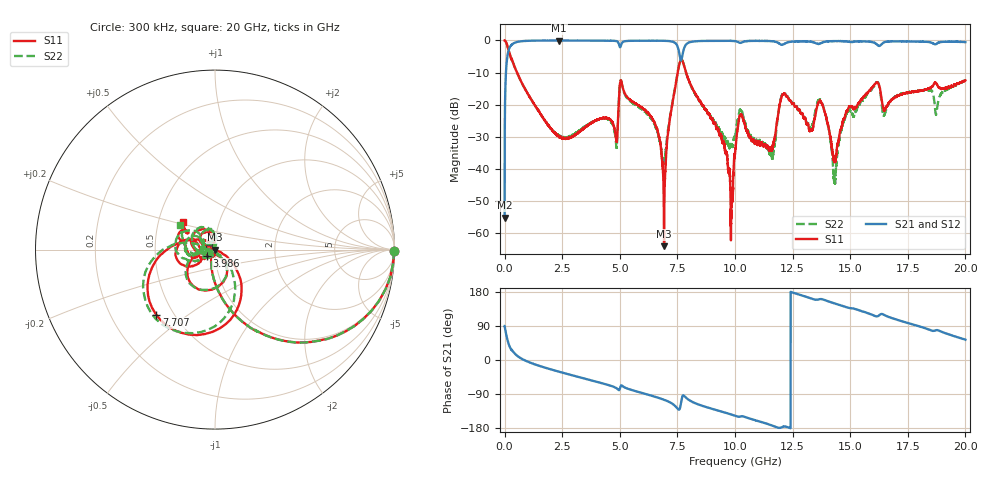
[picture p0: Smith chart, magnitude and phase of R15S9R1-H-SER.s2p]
!{R15S9R1}
!Johanson Technology Inc.
!www.johansontechnology.com
!Test Board Conditions:
!Substrate Type  RO4350B
!Substrate Thickness  20 mil
!Substrate Dk  3.66
!TL Type: GCPW
!TL Trace Width  34 mil
!TL Gap  10 mil
!Electrode orientation  Horizontal
!DUT TOPOLOGY	SERIES
!Mounting Pad LxW  26x52 mil
! Created Sat Feb  6 14:03:51 2021
# hz S ma R 50
! 2 Port Network Data from SP1.SP block
! freq  magS11  angS11  magS21  angS21  magS12  angS12  magS22  angS22
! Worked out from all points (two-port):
!   20001 points, 300 kHz to 20 GHz, reference 50 ohm
!   highest |S21| = -0.02 dB at 2.373 GHz (marker M1); lowest = -55.3 dB at 300 kHz (marker M2)
!   |S21| within 3 dB of the highest: 176.7 MHz to 7.556 GHz (7.379 GHz wide, 191 % of centre); 7.767 GHz to end of sweep
!   lowest |S11| = -64.2 dB at 6.923 GHz (marker M3), VSWR 1.00, Z = 50 - j0.0618 ohm
!   |S11| at or under -10 dB: 536 MHz to 7.515 GHz (6.979 GHz wide, 173 % of centre); 7.878 GHz to end of sweep
!   |S22| runs from -44.7 to 0.0 dB; largest |S21 - S12| = 0.014
!   S11 on the Smith chart (normalised r, x): 300 kHz: open; 3.986 GHz: 0.91, -0.06; 7.707 GHz: 0.40, -0.38; 20 GHz: 0.66, +0.22
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300000  1 -0.4  0.00172 89.6  0.001679 90.7  0.9977 -0.4
1.063e8  0.8541 -32.6  0.5154 57.2  0.5167 57.2  0.8544 -32.5
2.413e8  0.5836 -57.1  0.8062 32.5  0.8063 32.4  0.5846 -57.1
2.3733e9  0.03112 -123.9  0.998 -31.1  0.9971 -31.0  0.03172 -115.0
3.3343e9  0.04037 -135.0  0.9955 -46.8  0.9943 -46.8  0.04192 -135.0
3.9863e9  0.05687 -142.8  0.9922 -57.4  0.9925 -57.4  0.05707 -148.5
4.8223e9  0.03261 -134.1  0.9812 -73.2  0.9815 -73.2  0.02856 -140.9
5.0783e9  0.222 -131.8  0.8907 -67.0  0.8901 -67.0  0.2191 -137.2
6.6673e9  0.03496 168.7  0.9895 -99.7  0.9905 -99.6  0.03463 -176.8
6.9233e9  0.0006194 -85.9  0.9858 -105.1  0.9859 -105.0  0.01326 -101.8
7.7073e9  0.4895 -131.9  0.5588 -97.0  0.5617 -96.9  0.4932 -139.2
9.8203e9  0.002071 85.8  0.985 -143.5  0.9866 -143.5  0.02383 -148.1
1.00003e10  0.01765 -77.0  0.9749 -147.1  0.9764 -147.1  0.03219 -120.1
1.02613e10  0.06927 -164.3  0.9202 -148.6  0.9218 -148.6  0.08107 -174.3
1.15853e10  0.01967 168.0  0.9739 -172.2  0.9755 -172.2  0.01668 136.6
1.21133e10  0.1472 145.0  0.872 -175.6  0.8733 -175.7  0.1508 136.1
1.33343e10  0.04044 138.2  0.9492 161.8  0.95 161.8  0.04712 133.9
1.37583e10  0.1055 114.4  0.9156 160.6  0.9151 160.5  0.1083 105.1
1.43303e10  0.01294 169.2  0.9742 149.2  0.9782 149.1  0.006099 153.5
1.48993e10  0.08278 -142.7  0.9576 138.3  0.9584 138.2  0.07742 -150.7
1.66673e10  0.1065 -159.4  0.9653 113.7  0.9567 113.7  0.1032 -165.5
2e10  0.2391 139.5  0.9433 53.5  0.9362 53.2  0.2378 144.1
